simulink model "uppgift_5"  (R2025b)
settings: Solver=VariableStepAuto  StartTime=0.0  StopTime=10.0  RelTol=1e-3
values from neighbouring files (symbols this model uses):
  tau_d = 0.2    [Lektion_2.m]
  tau_mix = 0.14    [Lektion_2.m]
  tau_sensor = 0.05    [Lektion_2.m]

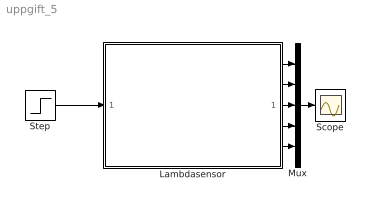
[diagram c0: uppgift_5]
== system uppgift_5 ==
  Lambdasensor : Subsystem
  Mux : Mux  Inputs=5
  Scope : Scope
  Step : Step  Time=5  Before=0.8  After=1.2  SampleTime=0
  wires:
  Lambdasensor/1(lambda_cyl [-]) -> Mux/1
  Lambdasensor/2(lambda_delay [-]) -> Mux/2
  Lambdasensor/3(lambda_eg [-]) -> Mux/3
  Lambdasensor/4(lambda_sensor [-]) -> Mux/4
  Lambdasensor/5(lambda_d [-]) -> Mux/5
  Mux/1 -> Scope/1
  Step/1 -> Lambdasensor/1(lambda_c [-])

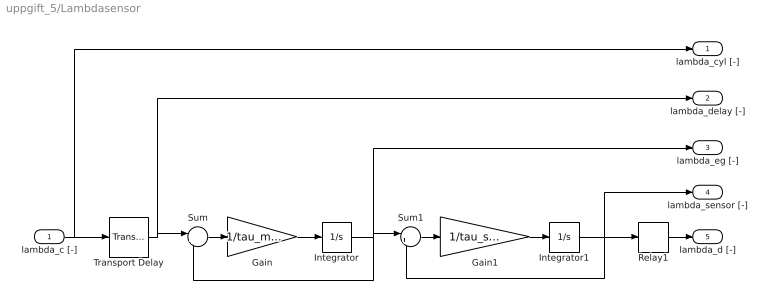
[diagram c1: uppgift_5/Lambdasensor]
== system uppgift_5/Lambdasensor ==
  lambda_c [-] : Inport
  Gain : Gain  Gain=1/tau_mix
  Gain1 : Gain  Gain=1/tau_sensor
  Integrator : Integrator  InitialCondition=0.8
  Integrator1 : Integrator  InitialCondition=0.8
  Relay1 : Relay  OnSwitchValue=1+eps  OffSwitchValue=1-eps
  Sum : Sum  Inputs=|+-
  Sum1 : Sum  Inputs=|+-
  Transport Delay : TransportDelay  DelayTime=tau_d  InitialOutput=0.8
  lambda_cyl [-] : Outport
  lambda_delay [-] : Outport  Port=2
  lambda_eg [-] : Outport  Port=3
  lambda_sensor [-] : Outport  Port=4
  lambda_d [-] : Outport  Port=5
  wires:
  lambda_c [-]/1 -> lambda_cyl [-]/1, Transport Delay/1
  Transport Delay/1 -> lambda_delay [-]/1, Sum/1
  Gain/1 -> Integrator/1
  Sum/1 -> Gain/1
  Integrator/1 -> Sum/2, lambda_eg [-]/1, Sum1/1
  Sum1/1 -> Gain1/1
  Gain1/1 -> Integrator1/1
  Integrator1/1 -> Relay1/1, Sum1/2, lambda_sensor [-]/1
  Relay1/1 -> lambda_d [-]/1
